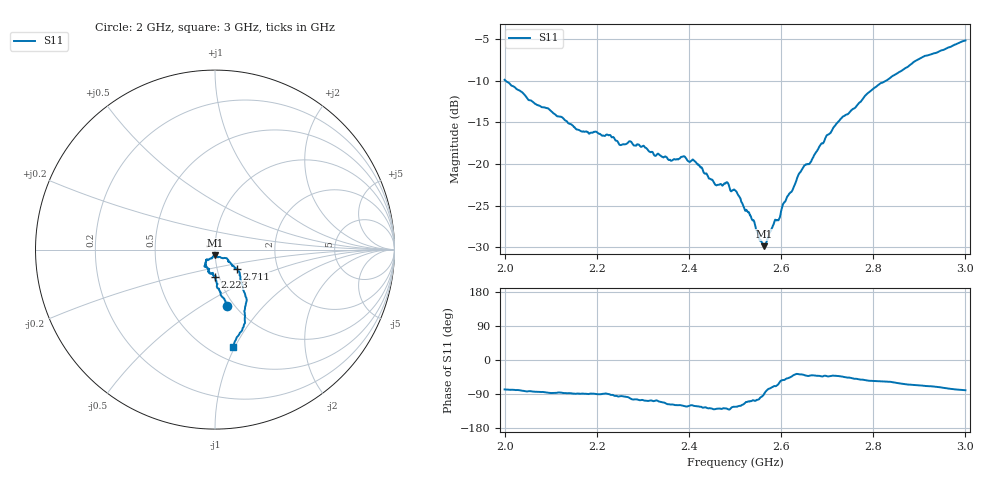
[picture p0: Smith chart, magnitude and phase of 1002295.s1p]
# Hz S DB R 50
! Planar, Obzor-804, 15045142, 19.1.3/3
! Date: 2/14/2023 4:18:03 PM
! Data: Format (Calibration Info)
! Freq	S11:dB/Ang(F1 Pxt)
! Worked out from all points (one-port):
!   2001 points, 2 GHz to 3 GHz, reference 50 ohm
!   lowest |S11| = -29.9 dB at 2.563 GHz (marker M1), VSWR 1.07, Z = 50 - j3.22 ohm
!   |S11| at or under -10 dB: 2.002 GHz to 2.828 GHz (826.4 MHz wide, 34.2 % of centre)
!   S11 on the Smith chart (normalised r, x): 2 GHz: 0.93, -0.65; 2.223 GHz: 0.96, -0.29; 2.711 GHz: 1.24, -0.27; 3 GHz: 0.63, -0.98
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2e9  -9.90 -77.7
2.0535e9  -12.35 -82.1
2.125e9  -14.41 -86.6
2.164e9  -16.01 -88.9
2.2225e9  -16.47 -89.3
2.25e9  -17.71 -95.7
2.273e9  -17.29 -101.6
2.3265e9  -19.03 -107.5
2.375e9  -19.43 -119.5
2.3875e9  -19.09 -120.8
2.4115e9  -19.61 -121.2
2.458e9  -22.50 -129.3
2.4815e9  -22.20 -128.0
2.5e9  -23.15 -123.3
2.538e9  -26.76 -106.5
2.555e9  -29.16 -99.0
2.5635e9  -29.86 -88.8
2.5955e9  -26.59 -61.1
2.6085e9  -24.53 -51.5
2.625e9  -23.10 -41.5
2.646e9  -20.60 -38.2
2.664e9  -19.78 -40.8
2.711e9  -15.90 -41.2
2.75e9  -13.68 -46.9
2.799e9  -11.01 -55.4
2.875e9  -8.34 -64.6
2.929e9  -6.77 -69.7
3e9  -5.18 -79.8
